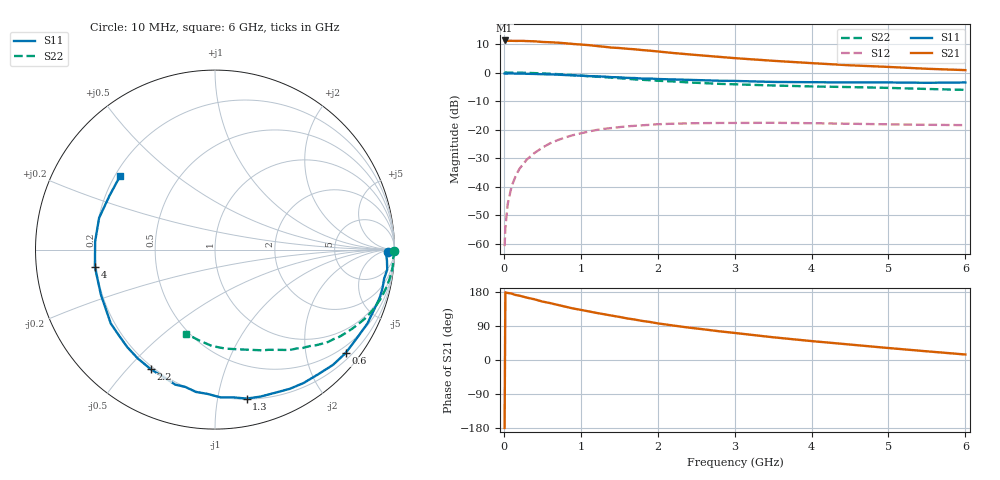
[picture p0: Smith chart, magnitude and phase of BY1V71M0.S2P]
! SIEMENS Small Signal Semiconductors
! BFY420
! Si NPN RF SIEGET Grounded Emitter Transistor in MICRO-X
! VCE = 1.75 V  IC = 1 mA
! Common Emitter S-Parameters:  October  1996
# GHz  S  MA  R  50
!  f  S11  S21  S12  S22
! GHz  MAG  ANG  MAG  ANG  MAG  ANG  MAG  ANG
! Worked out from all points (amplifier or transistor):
!   36 points, 10 MHz to 6 GHz, reference 50 ohm
!   highest |S21| = 11.2 dB at 10 MHz (marker M1)
!   |S21| within 3 dB of that: start of sweep to 1.649 GHz
!   unconditionally stable (mu >= 1): 4.55 GHz to end of sweep
!   at 250 MHz: K = 0.04, MSG = 21.6 dB, |S12| = -32.1 dB
!   at 1.4 GHz: K = 0.21, MSG = 14.1 dB, |S12| = -19.5 dB
!   at 6 GHz: K = 1.35, MAG = 6.1 dB, |S12| = -18.5 dB
!   S11 on the Smith chart (normalised r, x): 10 MHz: 46, -14; 600 MHz: 0.34, -2.84; 1.3 GHz: 0.20, -1.21; 2.2 GHz: 0.19, -0.58; 4 GHz: 0.19, -0.07; 6 GHz: 0.22, +0.33
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0.01  0.9612 -0.7  3.649 -179.3  0.0009 97.5  0.9999 -0.3
0.02  0.9538 -1.4  3.634 178.7  0.0019 80.2  0.9991 -0.6
0.05  0.9597 -3.5  3.594 176.9  0.0049 89.5  0.9972 -1.6
0.1  0.966 -6.6  3.599 175.3  0.01 88.5  0.9931 -3.3
0.15  0.9561 -9.8  3.582 171.7  0.0149 83.6  0.9946 -4.9
0.3  0.9498 -19.2  3.557 164.5  0.0299 78.5  0.9861 -9.7
0.4  0.9438 -25.9  3.526 160.1  0.0389 74.2  0.9762 -12.9
0.5  0.9317 -32.0  3.436 154.3  0.0481 70.4  0.9651 -16.1
0.6  0.9283 -38.4  3.393 150.2  0.0572 66.4  0.9502 -19.1
0.7  0.9191 -44.3  3.34 145.4  0.0652 63.0  0.9359 -22.0
0.9  0.8922 -56.4  3.167 136.0  0.0798 55.5  0.9001 -27.4
1.1  0.8645 -67.6  3.024 128.4  0.0921 49.4  0.8633 -32.6
1.3  0.8486 -78.0  2.834 120.9  0.1028 43.3  0.8283 -37.0
1.7  0.8002 -97.6  2.555 106.8  0.1161 33.0  0.7571 -45.1
2  0.7689 -110.8  2.34 96.7  0.1237 26.4  0.7172 -50.1
2.2  0.7564 -118.2  2.2 91.0  0.1266 22.5  0.6967 -53.4
2.8  0.7174 -138.5  1.88 75.8  0.1304 13.3  0.6329 -61.9
3.5  0.6833 -158.6  1.605 60.0  0.1312 5.8  0.5921 -70.6
4  0.6761 -171.7  1.461 49.9  0.1291 1.7  0.57 -77.0
4.5  0.6694 176.1  1.339 40.8  0.1263 -1.6  0.5551 -83.8
5.5  0.6601 152.9  1.163 22.9  0.1211 -4.4  0.5145 -99.6
6  0.669 142.3  1.101 14.5  0.1194 -4.2  0.4959 -108.7
